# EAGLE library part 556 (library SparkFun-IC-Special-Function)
556 Dual 555 timer 2 555 timers in one package 1MHZ 14DIP Datasheet SparkFun Products SparkFun SparkPunk Sound Kit (KIT-11177)
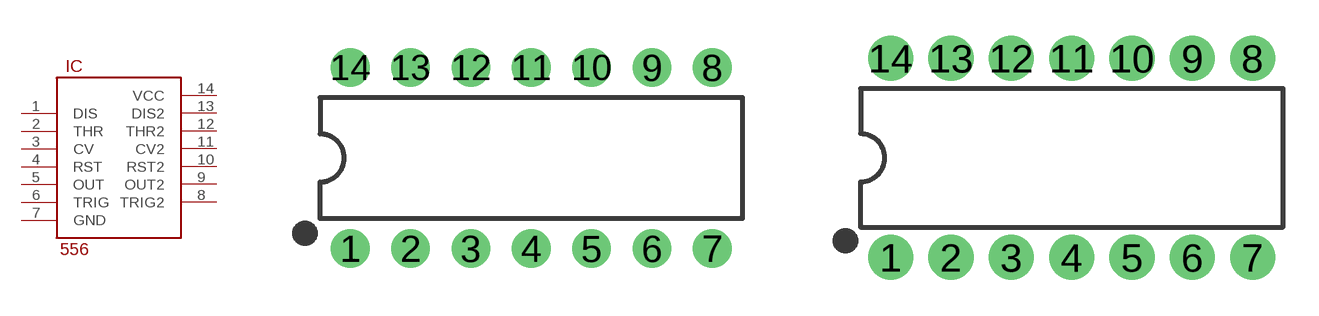
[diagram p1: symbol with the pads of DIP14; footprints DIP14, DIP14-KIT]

Designator prefix IC

## 556 (PROD_ID: IC-11898; VALUE: 556)  [DIP14]
1  DIS
2  THR
3  CV
4  RST
5  OUT
6  TRIG
7  GND
8  TRIG2
9  OUT2
10  RST2
11  CV2
12  THR2
13  DIS2
14  VCC

## 556KIT (PROD_ID: IC-11898; VALUE: 556)  [DIP14-KIT]
Pads as for DIP14

## Footprint DIP14 (pad centres in mm)
drill 0.813 pad 1.626: 1 -7.62,-3.81; 2 -5.08,-3.81; 3 -2.54,-3.81; 4 0,-3.81; 5 2.54,-3.81; 6 5.08,-3.81; 7 7.62,-3.81; 8 7.62,3.81; 9 5.08,3.81; 10 2.54,3.81; 11 0,3.81; 12 -2.54,3.81; 13 -5.08,3.81; 14 -7.62,3.81

## Footprint DIP14-KIT (pad centres in mm)
drill 0.864 pad 1.905: 1 -8.89,-4.191; 2 -6.35,-4.191; 3 -3.81,-4.191; 4 -1.27,-4.191; 5 1.27,-4.191; 6 3.81,-4.191; 7 6.35,-4.191; 8 6.35,4.191; 9 3.81,4.191; 10 1.27,4.191; 11 -1.27,4.191; 12 -3.81,4.191; 13 -6.35,4.191; 14 -8.89,4.191

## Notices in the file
Licensing: Creative Commons ShareAlike 4.0 International - https://creativecommons.org/licenses/by-sa/4.0
